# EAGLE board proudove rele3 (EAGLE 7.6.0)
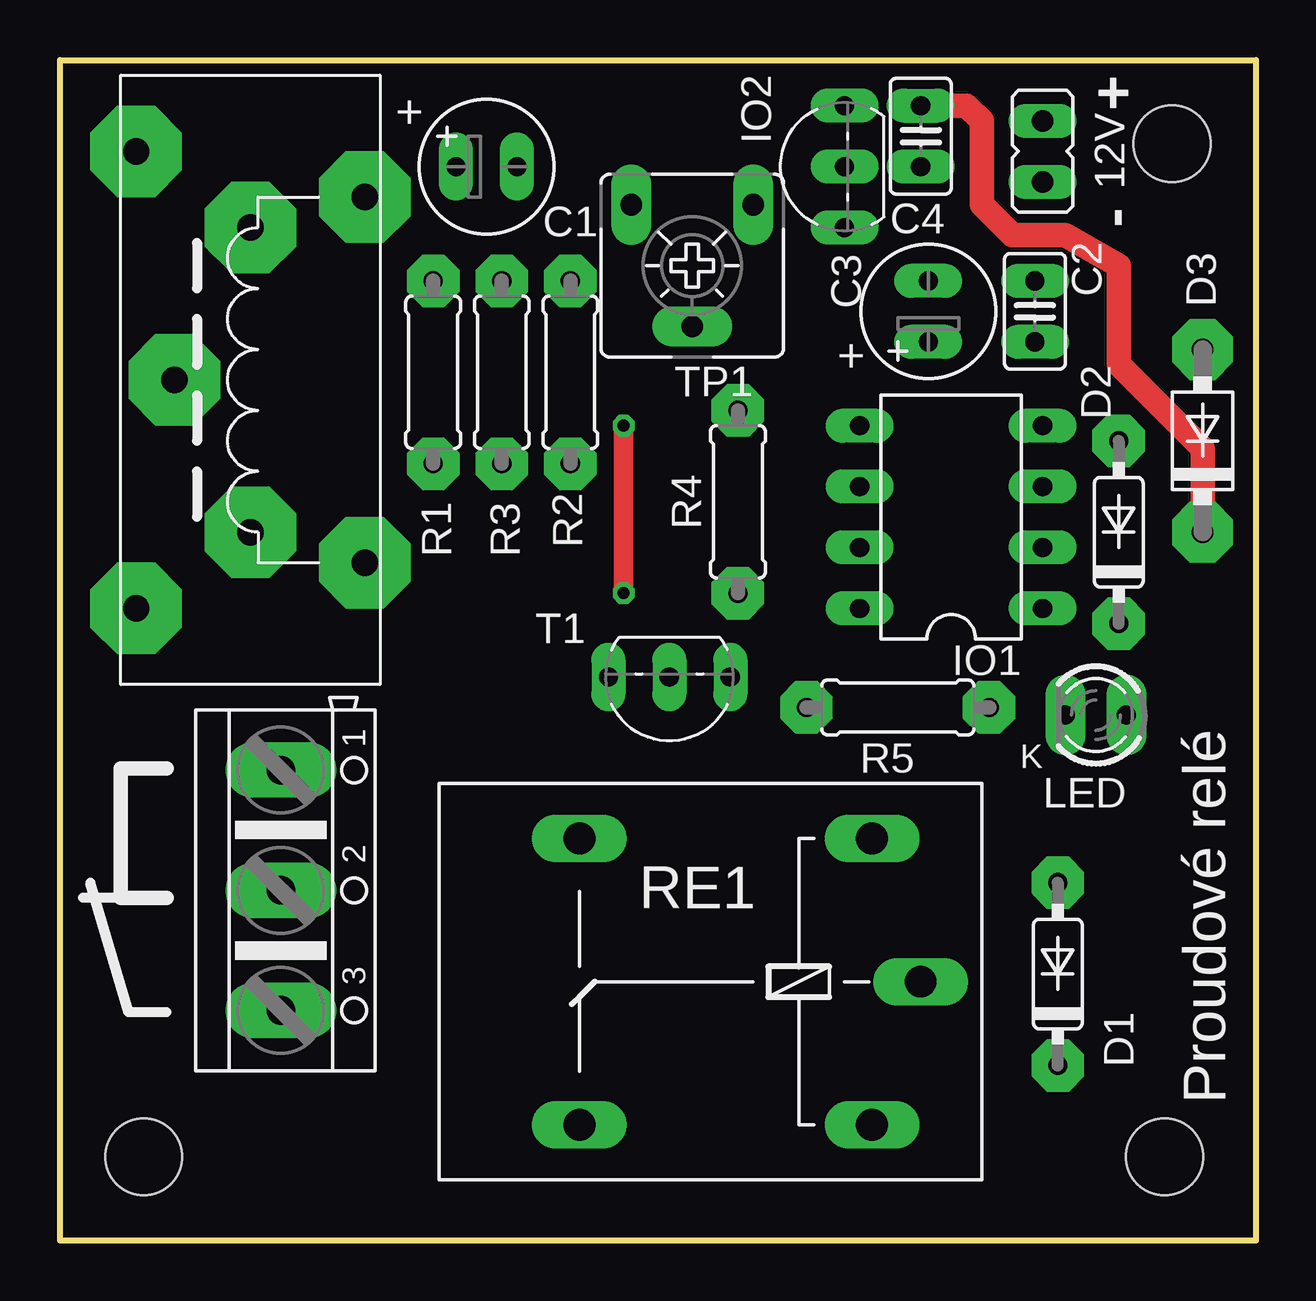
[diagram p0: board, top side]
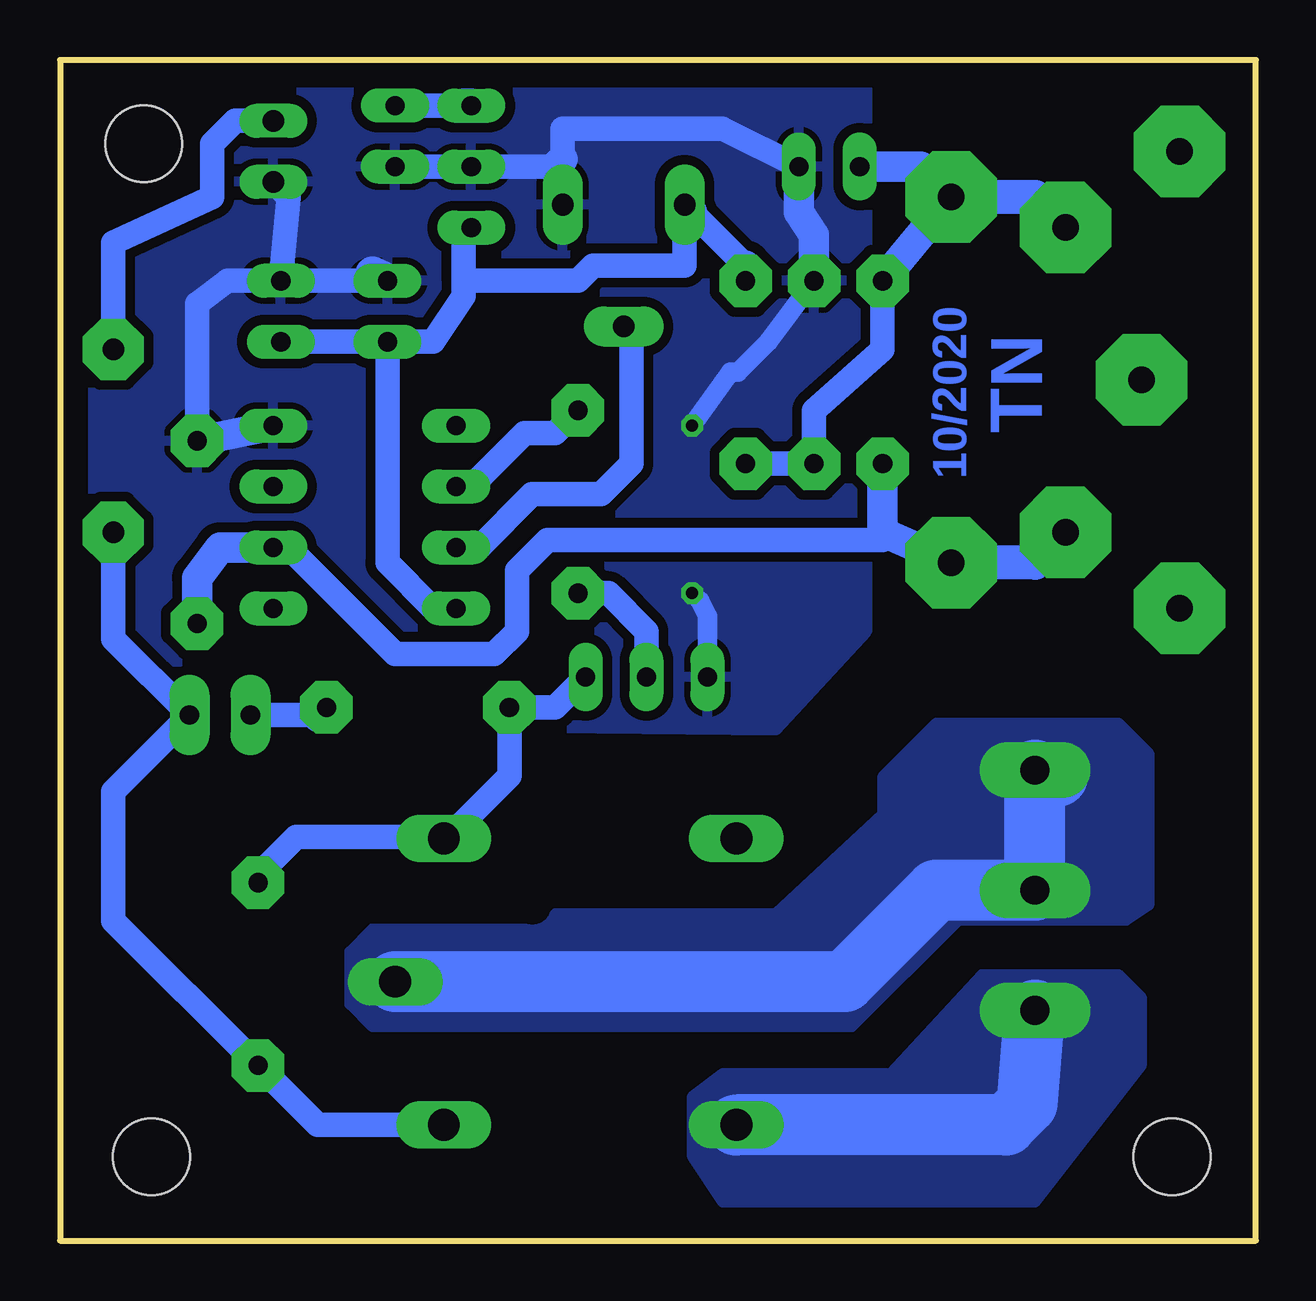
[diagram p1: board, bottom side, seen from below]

Size 49.85 x 49.21 mm. Coordinates in mm from the lower left corner, seen from the top.
Outline: 0,49.21 49.85,49.21 49.85,0 0,0 0,49.21
Copper layers (1*16): Top 0.035mm / dielectric 1.5mm / Bottom 0.035mm
Design rules "default": minimum track width 10mil, minimum drill 24mil, track to track 8mil, track to pad 8mil, pad to pad 8mil, via to via 8mil, smd to smd 8mil, copper to edge 40mil, drill to drill 8mil, minimum pad ring 10mil, minimum via ring 8mil, stop-mask expansion 4mil, vias tented up to drill 0mil, thermal gap 10mil
Holes 3.2 mm at 46.35,45.72 3.49,3.49 46.04,3.49

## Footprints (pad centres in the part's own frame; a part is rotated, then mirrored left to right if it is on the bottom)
JP1 = drill 0.9 pad 1.422 long: 1 0,-1.27; 2 0,1.27
E2,5-6 = drill 0.8 pad 1.422 long: + -1.27,0; - 1.27,0
C025-025X050 = drill 0.8 pad 1.422 long: 1 -1.27,0; 2 1.27,0
DO35-7 = drill 0.8 pad 2.184 octagon: A 3.81,0; C -3.81,0
DO41-7 = drill 0.9 pad 2.54 octagon: A 3.81,0; C -3.81,0
LSP11 = drill 1.1 pad 3.81 octagon: MP 0,0
AK500/3 = drill 1.2 pad 2.311 long: 1 -5.004,0; 2 0,0; 3 5.004,0
PROUDOVE_TRAFO = drill 1.1 pad 3.81 octagon: P$1 0,0; P$2 15.24,0; P$3 -1.905,9.525; P$4 17.145,9.525
DIL08 = drill 0.8 pad 1.422 long: 1 -3.81,-3.81; 2 -1.27,-3.81; 3 1.27,-3.81; 4 3.81,-3.81; 5 3.81,3.81; 6 1.27,3.81; 7 -1.27,3.81; 8 -3.81,3.81
TO92-CBE = drill 0.8 pad 1.422 long: B 0,0; C -2.54,0; E 2.54,0
LED3MM = drill 0.8 pad 1.676 long: A -1.27,0; K 1.27,0
0207/7 = drill 0.8 pad 2.184 octagon: 1 -3.81,0; 2 3.81,0
G5LE = drill 1.321 long: 1 -7.493,-5.969; 2 -7.493,5.969; O 4.699,5.969; P -9.525,0; S 4.699,-5.969
CA6V = drill 0.9 pad 1.676 long: A -2.54,-2.54; E 2.54,-2.54; S 0,2.54

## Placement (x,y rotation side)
12V  [JP1]  40.96,45.4 0 top
C1  47uF  [E2,5-6]  17.78,44.77 0 top
C2  100n  [C025-025X050]  40.64,38.73 270 top
C3  47uF  [E2,5-6]  36.2,38.73 90 top
C4  100n  [C025-025X050]  35.88,46.04 90 top
D1  1N4148  [DO35-7]  41.59,11.11 90 top
D2  5V1  [DO35-7]  44.13,29.53 90 top
D3  [DO41-7]  47.63,33.34 90 top
E$4  [LSP11]  7.94,29.53 0 top
E$5  [LSP11]  7.94,42.23 0 top
E$11  [AK500/3]  9.21,14.6 270 top
E$14  [PROUDOVE_TRAFO]  12.7,28.26 90 top
IO1  AttinyX5  [DIL08]  37.15,30.16 90 top
IO2  78L05  [TO92-CBE]  32.7,44.77 90 top
LED  [LED3MM]  43.18,21.91 180 top
R1  100R  [0207/7]  15.56,36.2 270 top
R2  100k  [0207/7]  21.27,36.2 90 top
R3  100k  [0207/7]  18.41,36.2 270 top
R4  1k  [0207/7]  28.26,30.8 90 top
R5  3k3  [0207/7]  34.93,22.23 0 top
RE1  [G5LE]  26.35,10.8 180 top
T1  BC337  [TO92-CBE]  25.4,23.49 180 top
TP1  50k  [CA6V]  26.35,40.64 180 top

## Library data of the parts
12V C1-C4 D1-D3 E$4 E$5 E$11 E$14 IO1 IO2 R1-R5 T1 TP1 = 11moje
LED = 10moje
RE1 = relay

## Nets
5V: C2.2 C3.+ IO1.8 IO2.C R2.2 TP1.E
AC1: E$11.1 E$11.2 RE1.P
AC2: E$11.3 RE1.O
GND: 12V.1 C1.- C2.1 C3.- C4.1 D2.A IO1.4 IO2.B R3.1 T1.E TP1.A
S$1: D1.A R5.1 RE1.1 T1.C
S$2: R4.1 T1.B
S$3: D2.C E$4.MP E$14.P$1 IO1.2 R1.2
S$4: IO1.6 R4.2
S$5: LED.K R5.2
S$6: C1.+ E$5.MP E$14.P$2 R1.1 R2.1 R3.2
S$7: 12V.2 D3.A
S$10: IO1.7 TP1.S
VIN: C4.2 D1.C D3.C IO2.E LED.A RE1.2

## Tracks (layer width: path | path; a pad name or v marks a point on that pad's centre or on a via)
5V
  Bottom 1.016: C3.+ C2.2 | C3.+ 34.29,37.46 33.02,39.37 33.02,40 | 33.02,40 33.02,41.91 | 33.02,40 28.26,40 27.62,40.64 23.81,40.64 23.81,42.54 23.49,42.86 21.27,40.64 | IO1.8 34.29,26.35 36.2,28.26 C3.+
  Bottom 1.27: 33.02,41.91 IO2.C | R2.2 21.27,40.64 | 23.49,42.86 TP1.E
AC1
  Bottom 2.54: RE1.P 17.15,10.8 13.34,14.6 E$11.2 E$11.1 8.26,19.37
  pour Bottom (no thermals): 37.78,12.06 36.83,13.02 30.48,13.02 arc-90 29.21,13.65 20,13.65 15.56,17.78 15.56,19.37 13.34,21.59 5.72,21.59 4.45,20.32 4.45,13.97 5.4,13.34 12.38,13.34 16.83,8.89 36.83,8.89 37.78,9.84
AC2
  Bottom 2.54: E$11.3 9.52,5.71 10.41,4.83 RE1.O
  pour Bottom (no thermals): 23.49,6.03 22.23,6.98 15.24,6.98 11.43,11.11 5.72,11.11 4.76,10.16 4.76,7.3 9.21,1.59 22.23,1.59 23.49,3.49
GND  (via drill 0.5)
  Top 0.813: v23.49,26.99 v23.49,33.97
  Bottom 0.813: R3.1 20.32,37.46 21.59,36.2 21.91,36.2 v23.49,33.97 | v23.49,26.99 23.18,26.67 22.86,26.03 T1.E
  Bottom 1.016: TP1.A 28.89,45.09 28.89,46.35 22.23,46.35 C1.- | C2.1 C3.- | C2.1 42.86,40 44.13,39.05 D2.A | C4.1 IO2.B 29.21,44.77 | C2.1 40.32,43.5 12V.1
  Bottom 1.27: C1.- 19.05,42.86 18.41,41.91 R3.1 | D2.A IO1.4 | 28.89,45.09 29.21,44.77
  Bottom 1.422: C3.- 36.83,40.32
  pour Bottom (isolate 0.406): 16.19,49.21 49.85,49.21 49.85,21.59 20,21.27 16.19,25.4
S$1
  Bottom 1.016: 41.59,15.24 40.01,16.83 33.66,16.83 | 33.72,16.76 31.12,19.37 R5.1 29.21,22.23 T1.C
  Bottom 1.422: 41.59,15.24 D1.A | 33.66,16.83 33.72,16.76 RE1.1
S$2
  Bottom 1.016: T1.B 25.4,25.4 26.99,26.99 R4.1
S$3
  Bottom 1.016: IO1.2 40.32,28.89 35.88,24.45 31.75,24.45 30.8,25.4 30.8,27.94 29.53,29.21 15.56,29.21 15.29,29.48 | 15.29,29.48 15.24,29.53 | 15.29,29.41 15.29,29.48
  Bottom 1.27: R1.2 15.56,29.53 15.29,29.41 E$14.P$1 | D2.C 44.13,27.62 43.18,28.89 IO1.2
  Bottom 1.422: E$14.P$1 9.21,28.26 E$4.MP
S$4
  Bottom 1.016: IO1.6 32.7,31.43 30.48,33.66 29.21,33.66 R4.2
S$5
  Bottom 1.016: 39.05,21.91 LED.K
  Bottom 1.422: R5.2 39.05,21.91
S$6
  Bottom 1.016: R1.1 15.56,37.15 18.41,34.61 R3.2 R2.1
  Bottom 1.27: C1.+ 13.97,44.77 E$14.P$2 R1.1
  Bottom 1.422: E$14.P$2 9.21,43.5 E$5.MP
S$7
  Bottom 1.016: D3.A 47.63,41.59 43.5,43.5 43.5,45.72 42.55,46.67 12V.2
S$9  (via drill 1.1 pad 3.81)
  other vias: 4.76,35.88
S$10
  Bottom 1.016: IO1.7 32.38,28.89 30.16,31.12 27.3,31.12 26.04,32.38 26.04,37.78 TP1.S
VIN
  Top 1.016: D3.C 47.63,33.02 44.13,36.51 44.13,40.64 41.91,41.91 39.69,41.91 38.42,43.18 38.42,46.67 37.78,47.31 C4.2
  Bottom 1.016: RE1.2 39.12,4.83 D1.C 47.63,13.34 47.63,18.73 LED.A 47.63,25.08 D3.C | C4.2 IO2.E
  Bottom 1.422: IO2.E 33.02,47.31

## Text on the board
Bottom: TN | 10/2020
tPlace: + | + | K
tNames: + | - | Proudové relé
